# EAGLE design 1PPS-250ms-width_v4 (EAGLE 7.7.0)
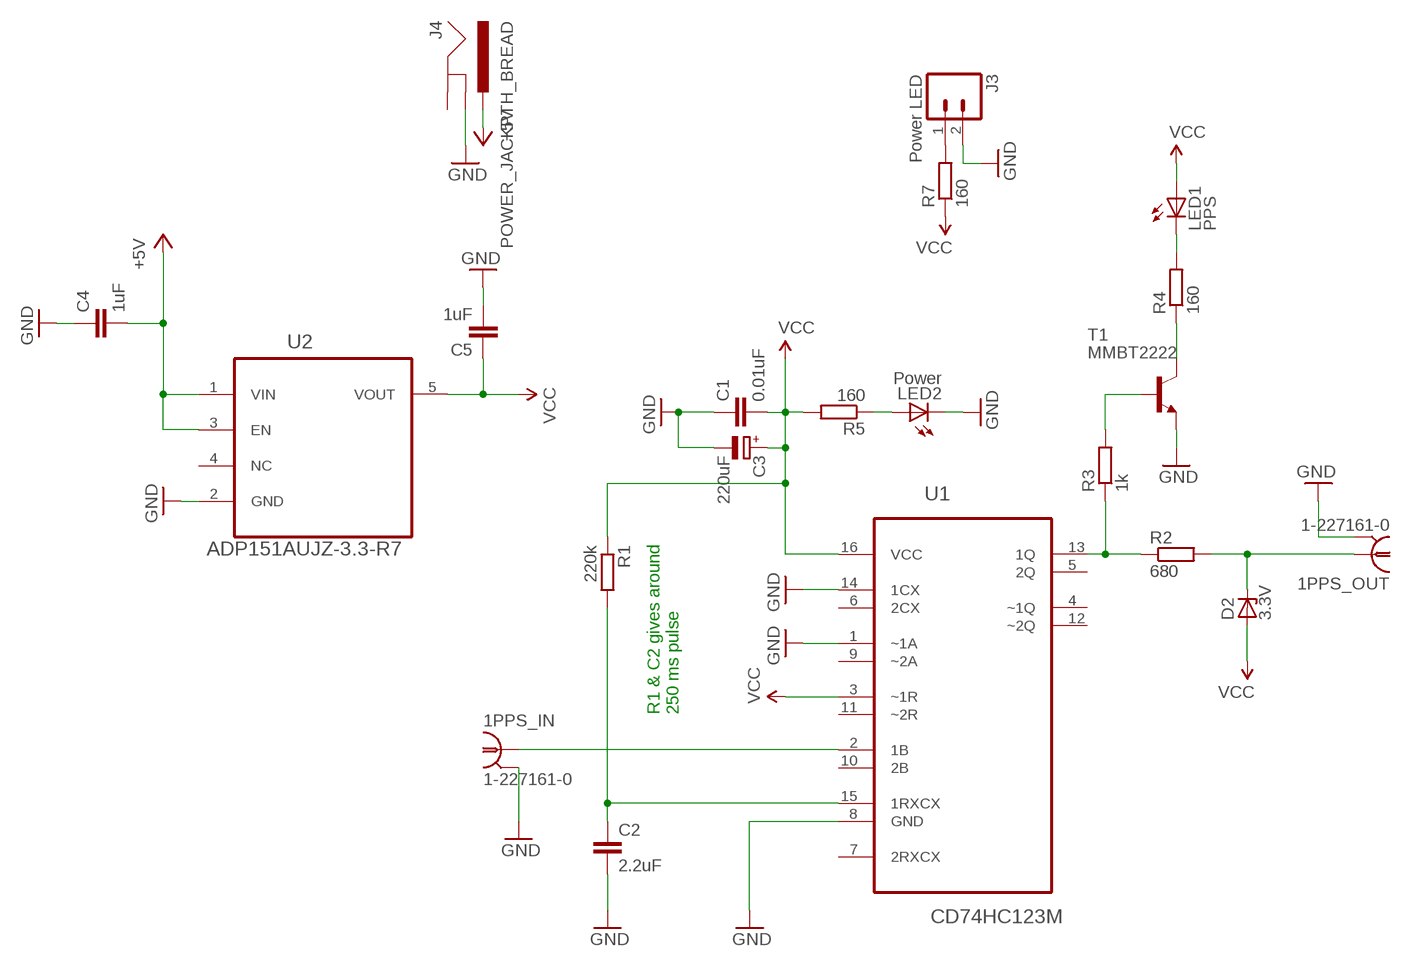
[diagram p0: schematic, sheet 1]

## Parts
1PPS_IN  1-227161-0  [AMP_227161]
1PPS_OUT  1-227161-0  [AMP_227161]
C1  0.01uF  C-EUC1206  [C1206]
C2  2.2uF  C-EUC1206  [C1206]
C3  220uF  CPOL-EU140CLH-1010  [140CLH-1010]
C4  1uF  C-EUC1206  [C1206]
C5  1uF  C-EUC1206  [C1206]
D2  3.3V  ZENER-DIODE  [SOD123]
J3  Power LED  M02PTH  [1X02]
J4  POWER_JACKPTH_BREAD  [POWER_JACK_PTH_BREAD]
LED1  PPS  LEDCHIPLED_0603  [CHIPLED_0603]
LED2  Power  LEDCHIPLED_0603  [CHIPLED_0603]
R1  220k  R-EU_R0805  [R0805]
R2  680  R-EU_R0805  [R0805]
R3  1k  R-EU_R0805  [R0805]
R4  160  R-EU_R0805  [R0805]
R5  160  R-EU_R0805  [R0805]
R7  160  R-EU_R0805  [R0805]
T1  MMBT2222  MMBT2222ALT1-NPN-SOT23-BEC  [SOT23-BEC]
U1  CD74HC123M  [SOIC127P600X175-16N]
U2  ADP151AUJZ-3.3-R7  [SOT95P280X100-5N]

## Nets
+5V: C4.2 J4.PWR U2.1(VIN) U2.3(EN)
GND: 1PPS_IN.2 1PPS_OUT.2 C1.1 C2.2 C3.- C4.1 C5.2 J3.2 J4.GNDBREAK LED2.C T1.E U1.1(~1A) U1.8(GND) U1.14(1CX) U2.2(GND)
N$1: 1PPS_IN.1 U1.2(1B)
N$2: R2.1 R3.1 U1.13(1Q)
N$3: C2.1 R1.2 U1.15(1RXCX)
N$4: 1PPS_OUT.1 D2.C R2.2
N$6: R3.2 T1.B
N$7: R4.1 T1.C
N$8: LED1.C R4.2
N$9: LED2.A R5.1
N$11: J3.1 R7.2
VCC: C1.2 C3.+ C5.1 D2.A LED1.A R1.1 R5.2 R7.1 U1.3(~1R) U1.16(VCC) U2.5(VOUT)
Unconnected: J4.GND U1.4(~1Q) U1.5(2Q) U1.6(2CX) U1.7(2RXCX) U1.9(~2A) U1.10(2B) U1.11(~2R) U1.12(~2Q) U2.4(NC)

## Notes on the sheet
- R1 & C2 gives around
  250 ms pulse

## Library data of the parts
1PPS_IN 1PPS_OUT = con-coax:?227161*: JACK, RIGHT ANGLE, 50 OHM, PCB, BNC; MF: TYCO ELECTRONICS; MPN: 1-227161; OC_FARNELL: unknown; OC_NEWARK: 33B3200
C1 C4 C5 = resistor:C-EU: CAPACITOR, European symbol
C2 = rcl:C-EU: CAPACITOR, European symbol
C3 = rcl:CPOL-EU: POLARIZED CAPACITOR, European symbol
D2 = jackens:ZENER-DIODE: Z-Diode
J3 = SparkFun-Connectors:M02: Standard 2-pin 0.1" header. Use with
J4 = SparkFun-Connectors:POWER_JACK: Power Jack This is the standard 5.5mm barrel jack for power. The PTH is the most common, proven, reliable, footprint. The Slot footprint only works if the mill layer is transmitted to the PCB fab house so be warned. Mating wall wart : TOL-00298 (and others); PROD_ID: PRT-10811
LED1 LED2 = adafruit:LED: LED
R1-R5 R7 = resistor:R-EU_: RESISTOR, European symbol
T1 = transistor:*-NPN-: NPN Transistror BF959 corrected 2008.03.06
U1 = Texas Instruments_By_element14_Batch_1:CD74HC123M: High-Speed CMOS Logic Dual Retriggerable Monostable Multivibrators with Resets; MPN: CD74HC123M; OC_FARNELL: 1103157; OC_NEWARK: 34K2410; PACKAGE: SOIC-16; SUPPLIER: Texas Instruments
U2 = Analog Devices_By_element14_Batch_1:ADP151AUJZ-3.3-R7: Ultralow Noise,200 mA, CMOS Linear Regulator; MPN: ADP151AUJZ-3.3-R7; OC_FARNELL: -; OC_NEWARK: 74R5887; PACKAGE: TSOT-5; SUPPLIER: Analog Devices

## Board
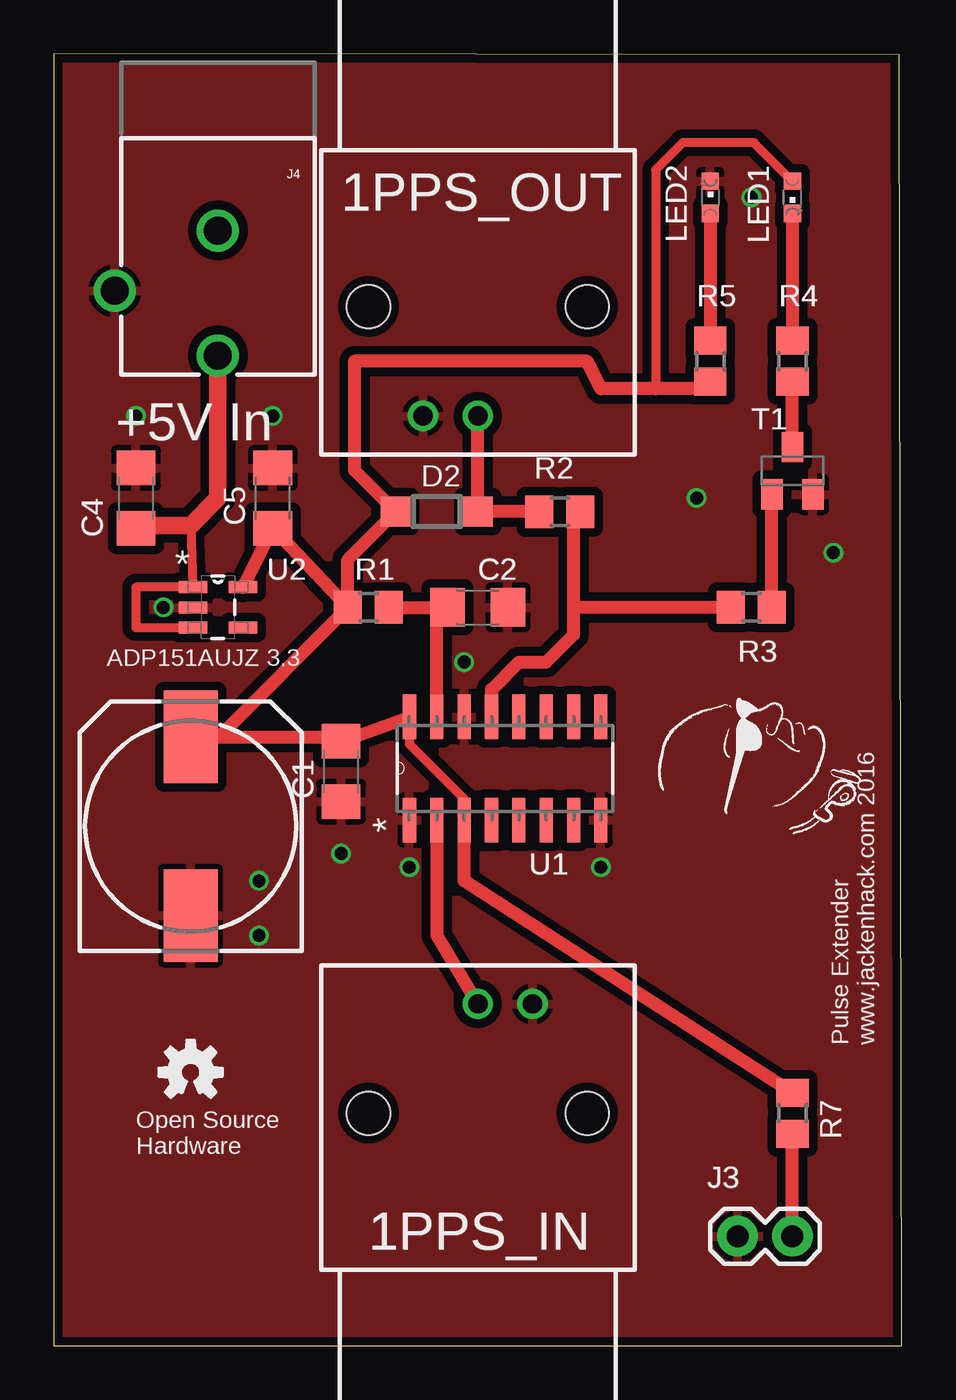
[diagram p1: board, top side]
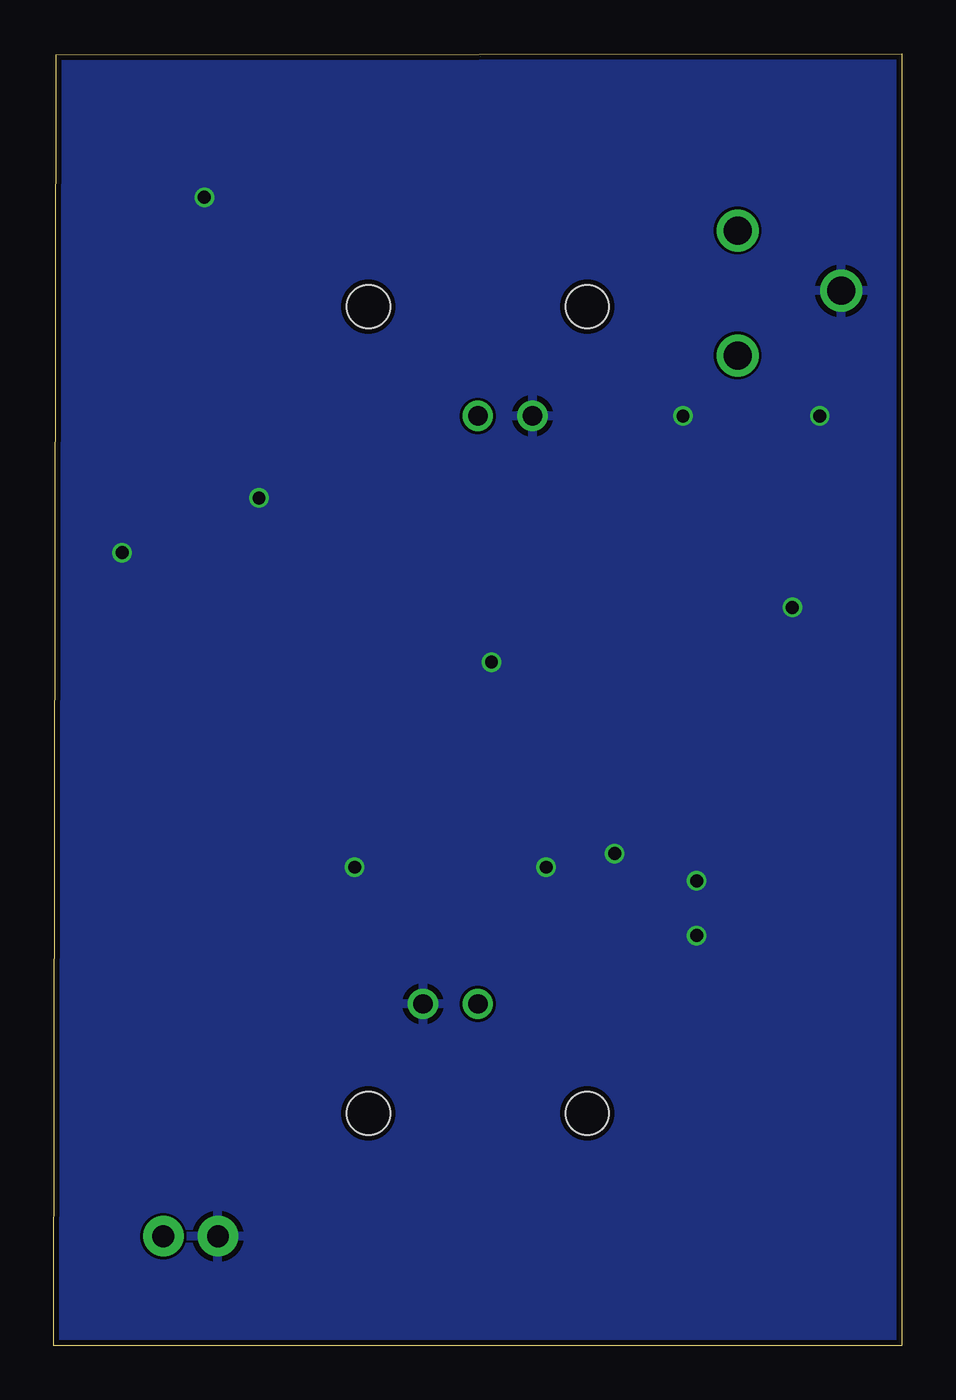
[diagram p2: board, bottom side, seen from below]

Size 39.37 x 60 mm. Coordinates in mm from the lower left corner, seen from the top.
Outline: 0,60 0,0 39.37,0 39.25,59.97 0,60
Copper layers (1*16): Top 0.035mm / dielectric 1.5mm / Bottom 0.035mm
Design rules "dirt_cheap_dirty_boards.v1": minimum track width 5mil, minimum drill 12mil, track to track 5mil, track to pad 5mil, pad to pad 5mil, via to via 5mil, smd to smd 0mil, copper to edge 10mil, drill to drill 10mil, minimum pad ring 10mil, minimum via ring 6mil, stop-mask expansion 2mil, vias tented up to drill 25mil, thermal gap 10mil

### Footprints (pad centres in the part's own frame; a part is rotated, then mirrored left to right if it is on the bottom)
AMP_227161 = drill 0.9 pad 1.27: 1 0,-5.08; 2 -2.54,-5.08 | hole 2: -5.08,0; 5.08,0
C1206 = smd 1.6 x 1.8: 1 -1.4,0; 2 1.4,0
140CLH-1010 = smd 4.3 x 2.5: + 4.15,0; - -4.15,0
SOD123 = smd 1.4 x 1.4: A 1.9,0; C -1.9,0
1X02 = drill 1.016 pad 1.88: 1 0,0; 2 2.54,0
POWER_JACK_PTH_BREAD = drill 1.3: GND 0,7.9; GNDBREAK 4.8,10.7; PWR 0,13.7
CHIPLED_0603 = smd 0.8 x 0.8: A 0,-0.75; C 0,0.75
R0805 = smd 1.3 x 1.5: 1 -0.95,0; 2 0.95,0
SOT23-BEC = smd 1 x 1.4: B -0.95,-1.1; C 0,1.1; E 0.95,-1.1
SOIC127P600X175-16N = smd 2.057 x 0.61: 1 -4.801,8.89; 2 -4.801,7.62; 3 -4.801,6.35; 4 -4.801,5.08; 5 -4.801,3.81; 6 -4.801,2.54; 7 -4.801,1.27; 8 -4.801,0; 9 0,0; 10 0,1.27; 11 0,2.54; 12 0,3.81; 13 0,5.08; 14 0,6.35; 15 0,7.62; 16 0,8.89
SOT95P280X100-5N = smd 1.321 x 0.559: 1 -1.168,0.94; 2 -1.168,0; 3 -1.168,-0.94; 4 1.168,-0.94; 5 1.168,0.94

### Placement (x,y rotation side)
1PPS_IN  19.68,10.79 180 top
1PPS_OUT  19.68,48.26 0 top
C1  13.34,26.67 90 top
C2  19.68,34.29 0 top
C3  6.35,24.13 90 top
C4  3.81,39.37 270 top
C5  10.16,39.37 90 top
D2  17.78,38.73 180 top
J3  34.29,5.08 180 top
J4  7.62,59.69 180 top
LED1  34.29,53.34 180 top
LED2  30.48,53.34 0 top
R1  14.61,34.29 0 top
R2  23.5,38.73 180 top
R3  32.38,34.29 0 top
R4  34.29,45.72 90 top
R5  30.48,45.72 270 top
R7  34.29,10.79 270 top
T1  34.29,40.64 0 top
U1  25.4,29.21 90 top
U2  7.62,34.29 0 top
U$1  [OSHW-LOGO-S]  6.35,12.7 0 top

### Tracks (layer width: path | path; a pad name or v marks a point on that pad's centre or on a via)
+5V
  Top 0.406: 6.35,38.1 U2.1 3.81,35.23 3.81,33.35 U2.3
  Top 0.813: J4.PWR 7.62,39.37 6.35,38.1 3.94,38.1 C4.2
GND  (via drill 0.6)
  other vias: 19.05,31.75 32.38,53.34 25.4,22.23 3.81,43.18 13.34,22.86 9.53,21.59 16.51,22.23 10.16,43.18 9.53,19.05 5.08,34.29 29.84,39.37 36.2,36.83
  pour Top (isolate 0.406): 0,60.96 39.37,60.96 39.37,-1.27 0,-1.27
  pour Bottom: 0,60.96 39.37,60.96 39.37,-1.27 0,-1.27
N$1
  Top 0.61: U1.2 17.78,19.05 1PPS_IN.1
N$2
  Top 0.61: U1.13 20.32,30.48 21.59,31.75 22.86,31.75 24.13,33.02 24.13,34.29 | 24.13,34.29 24.13,38.42 R2.1 | R3.1 24.13,34.29
N$3
  Top 0.61: U1.15 17.78,33.78 C2.1 R1.2
N$4
  Top 0.61: R2.2 D2.C 1PPS_OUT.1
N$6
  Top 0.61: R3.2 T1.B
N$7
  Top 0.61: T1.C R4.1
N$8
  Top 0.61: LED1.C R4.2
N$9
  Top 0.61: LED2.A R5.1
N$11
  Top 0.61: J3.1 R7.2
VCC
  Top 0.406: LED1.A 32.5,55.88 29.21,55.88 27.94,54.61 27.94,44.45 | U1.16 16.51,27.94 19.05,25.4 U1.3
  Top 0.61: U2.5 C5.1 R1.1 | U1.16 C1.2 13.12,28.28 7.64,28.28 | R1.1 13.65,36.51 D2.A 13.97,40.65 13.97,45.72 24.77,45.72 25.4,44.45 27.94,44.45 30.16,44.45 R5.2 | R7.1 19.05,21.59 U1.3 | C3.+ 7.64,28.28 | 7.64,28.28 R1.1

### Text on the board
tPlace: +5V In | Pulse Extender / www.jackenhack.com 2016 | Open Source / Hardware
tNames: ADP151AUJZ 3.3
_tNames: J4 | LED1 | 1PPS_OUT | LED2 | R5 | R4 | T1 | D2 | R2 | C4 | C5 | U2 | R1 | C2 | R3 | C1 | U1 | R7 | J3 | 1PPS_IN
